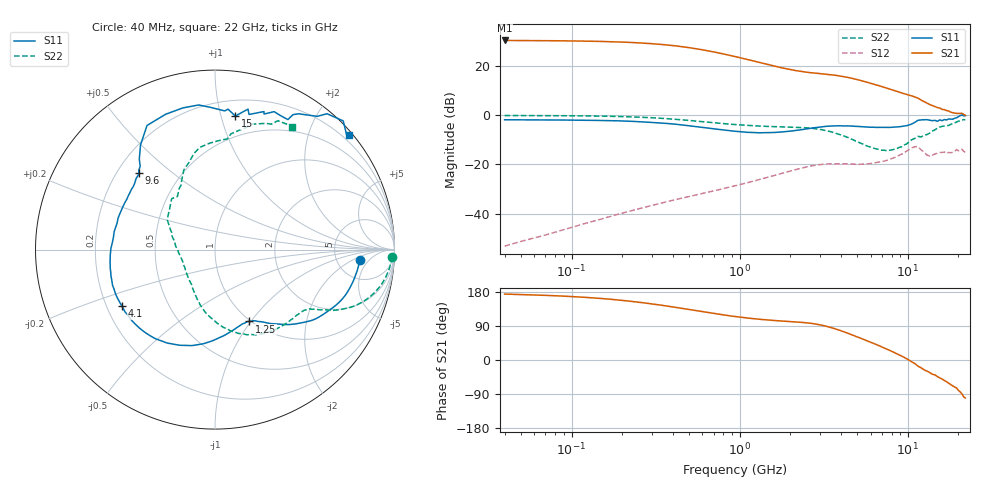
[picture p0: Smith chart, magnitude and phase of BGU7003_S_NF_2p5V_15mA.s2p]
!	Filename:	P:\Prog\Test\Noise\ATS_data\Testdata_Net\BGU7002	BGU7003	RN20082092\BGU7003_B1_high	freq_bias	loop_2.53V13.6mA_D.s2p
!	Date/Time:	Tue	16-Sep-08	9:24:09
!	BGU7003_B1_high	freq_bias	loop
!	bias	mode	1:00	Vout=	2.529	"V,"	Iout=13.5850	"mA,"	Vin=	5.915	"V,"	Iin=	1.449	mA
!	Date/time	Mon	Aug	11	1:45:17	2008
!	Device	data	file	deembeded	for	feedlines	and	parallel
!	Original	file:	\BGU7002	BGU7003	RN20082092\BGU7003_B1_high	freq_bias	loop_2.53V13.6mA_R.s2p
!	Feed-files:	PR029V01_high	"frequency_140808_Feed1.s2p,"	PR029V01_high	frequency_140808_Feed2.s2p
!	Parallel-file:	PR029V01_high	frequency_140808_Par.s2p
#	MHz	S	MA	R	50
!	Freq-MHz	S11-mag	S11-arg	S21-mag	S21-arg	S12-mag	S12-arg	S22-mag	S22-arg
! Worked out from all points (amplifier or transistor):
!   160 points, 40 MHz to 22 GHz, reference 50 ohm
!   highest |S21| = 30.3 dB at 40 MHz (marker M1)
!   |S21| within 3 dB of that: start of sweep to 509.8 MHz
!   unconditionally stable (mu >= 1): nowhere
!   at 300 MHz: K = 0.33, MSG = 32.8 dB, |S12| = -36.6 dB
!   at 2.25 GHz: K = 0.62, MSG = 19.8 dB, |S12| = -21.7 dB
!   at 22 GHz: K = -0.01, MSG = 7.5 dB, |S12| = -15.0 dB
!   lowest NFmin = 0.69 dB at 400 MHz
!   S11 on the Smith chart (normalised r, x): 40 MHz: 8.55, -2.78; 1.25 GHz: 0.99, -0.98; 4.1 GHz: 0.26, -0.26; 9.6 GHz: 0.29, +0.39; 15 GHz: 0.32, +1.11; 22 GHz: 0.07, +2.70
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40  0.8088 -4.0  32.9 174.0  0.0022 75.8  0.9862 -2.3
70  0.8032 -7.2  32.5 170.6  0.00371 79.5  0.9815 -4.6
120  0.7909 -12.5  31.89 165.4  0.00634 80.1  0.9694 -8.0
160  0.7793 -16.5  31.25 161.4  0.00835 79.0  0.9549 -10.6
210  0.7605 -21.3  30.3 156.3  0.01075 77.6  0.9337 -13.6
270  0.7293 -26.6  29.01 150.7  0.01346 75.6  0.905 -16.7
330  0.6989 -31.6  27.59 145.6  0.01603 73.9  0.8734 -19.4
420  0.6539 -37.8  25.45 138.6  0.01954 71.7  0.8242 -22.9
550  0.5883 -45.2  22.36 130.1  0.02412 69.6  0.7614 -26.2
700  0.5295 -51.3  19.27 122.8  0.02909 68.0  0.7037 -28.5
950  0.4713 -58.3  15.36 114.5  0.0373 66.3  0.645 -31.0
1250  0.4431 -64.5  12.24 108.3  0.04744 64.1  0.607 -33.6
1900  0.466 -79.5  8.74 102.1  0.07013 56.5  0.5779 -42.2
2700  0.5501 -103.5  7.256 96.4  0.09426 42.9  0.5428 -59.2
3500  0.6045 -130.6  6.634 85.5  0.1036 29.4  0.4604 -79.3
4100  0.6062 -148.7  6.109 75.4  0.103 23.6  0.385 -92.5
5600  0.5797 179.2  4.766 52.4  0.1016 19.9  0.2445 -121.4
7800  0.5658 150.5  3.399 25.4  0.1269 21.0  0.1946 -166.4
9600  0.6022 134.8  2.715 6.0  0.1778 14.1  0.2525 161.8
11500  0.7884 118.7  2.221 -16.4  0.2293 -20.7  0.3725 130.4
15000  0.7526 81.4  1.431 -43.9  0.1683 -29.8  0.5487 102.3
22000  0.9829 40.6  0.9921 -100.5  0.1775 -80.9  0.8052 58.0
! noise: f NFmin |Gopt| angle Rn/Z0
400  0.687  0.139  14.05  0.115
1000  0.784  0.146  30.72  0.127
1500  0.865  0.152  44.61  0.133
1700  0.897  0.155  50.16  0.134
2200  0.978  0.162  64.06  0.135
3000  1.107  0.177  86.28  0.131
4400  1.333  0.208  125.2  0.116
5800  1.559  0.248  164.1  0.102
8000  1.915  0.326  -152.9  0.115
1.2e+04  2.561  0.519  -111.3  0.399
